FUNCTION_BLOCK Example33_StarWheel //3x3 flyways 6 xbots - star wheel module demo CreateStar, DeleteStar, GetStarStatus, SendXbotToStar, StarExitClear
VAR_INPUT
	Execute : BOOL;
END_VAR
VAR_OUTPUT
END_VAR
VAR_IN_OUT
	PM_Controller : PMControllerType;	// the planar motor controller to use
END_VAR
VAR
	Setup : Example33_StarWheelSetup;
	wheel_angle : REAL;
	write_angle : PMC_WriteStream;	
	rotation_speed : REAL := 1.0;
	next_xbot : USINT := 1;
	
	check_wheel_status : PMC_Star_GetStarStatus;
	execute_return : BOOL;
	return_xbot : PMC_RunMacro;
	clear_exit : PMC_Star_StarExitClear;
	
	read_xbot_state : PMC_ReadXbotState;
	next_xbot_ready : BOOL;
	send_xbot_to_wheel : PMC_Star_SendXbotToStar;
END_VAR
VAR CONSTANT
	PI : REAL := 3.141593;
	cycle_time : REAL := 0.001;
END_VAR

//3x3 flyways 6 xbots - star wheel module demo CreateStar, DeleteStar, GetStarStatus, SendXbotToStar, StarExitClear

//reset wheel angle
IF(NOT(Setup.Done))THEN
	wheel_angle := 0;
	next_xbot := 1;
END_IF;

//Initial setup
Setup(Execute := Execute,PM_Controller := PM_Controller);

//check if xbot is in exit, if it is return it to queue and clear the star wheel's exit
check_wheel_status(Execute := Setup.Done AND NOT(check_wheel_status.Done),WheelID := 1,PM_Controller := PM_Controller); 
IF(check_wheel_status.Done AND check_wheel_status.ExitState = 1)THEN
	execute_return := TRUE;
END_IF;
return_xbot(Execute := execute_return,cmdLB := 0,MacroID := 128,XbotID := check_wheel_status.ExitXID,PM_Controller := PM_Controller);
clear_exit(Execute := return_xbot.Ack,WheelID := 1,PM_Controller := PM_Controller);
IF(clear_exit.Done)THEN
	execute_return := FALSE;
END_IF;

//check if next xbot in queue is ready to go, if it is send it to the star wheel
read_xbot_state(Enable := Setup.Done,XbotID := next_xbot,PM_Controller := PM_Controller);
IF(read_xbot_state.State = 3)THEN
	next_xbot_ready := TRUE;
END_IF;
send_xbot_to_wheel(Execute := next_xbot_ready,WheelID := 1,XbotID := next_xbot,PM_Controller := PM_Controller);
IF(send_xbot_to_wheel.Done)THEN
	next_xbot := next_xbot + 1;
	IF(next_xbot > 6)THEN
		next_xbot := 1;
	END_IF;
	next_xbot_ready := FALSE;
END_IF;

//write wheel angle
write_angle(Enable := TRUE,StmID := 1,AxisID := 6,Pos := wheel_angle,PM_Controller := PM_Controller);
	
//increment wheel angle
wheel_angle := wheel_angle + rotation_speed*cycle_time;

//2PI wrap around handling
IF(wheel_angle > 2*PI)THEN
	wheel_angle := wheel_angle - 2*PI;
END_IF;

END_FUNCTION_BLOCK
